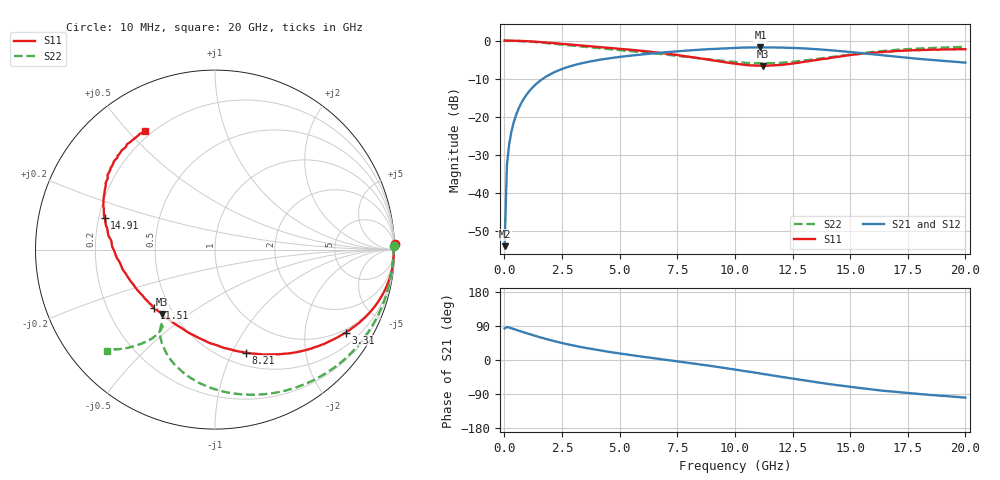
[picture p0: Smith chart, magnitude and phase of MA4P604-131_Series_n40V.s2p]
! AWR Design Environment (9226) Thu Aug 19 15:08:55 2021
! Document = 'n40V'
! nPorts: 2, nXvals: 201
# GHz S DB R 50
!Freq DBS11 AngS11 DBS21 AngS21 DBS12 AngS12 DBS22 AngS22
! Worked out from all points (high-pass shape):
!   201 points, 10 MHz to 20 GHz, reference 50 ohm
!   highest |S21| = -1.79 dB at 11.11 GHz (marker M1); lowest = -54.1 dB at 10 MHz (marker M2)
!   |S21| within 3 dB of the highest: 4.42 GHz to 17.94 GHz (13.52 GHz wide, 121 % of centre)
!   lowest |S11| = -6.7 dB at 11.21 GHz (marker M3), VSWR 2.73, Z = 21.7 - j20 ohm
!   |S11| at or under -10 dB: nowhere
!   |S22| runs from -6.0 to 0.0 dB; largest |S21 - S12| = 0.024
!   S11 on the Smith chart (normalised r, x): 10 MHz: -5, +62; 3.31 GHz: 0.89, -3.21; 8.21 GHz: 0.63, -1.13; 11.51 GHz: 0.41, -0.34; 14.91 GHz: 0.22, +0.13; 20 GHz: 0.17, +0.56
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0.01  0.02 1.8  -54.08 83.3  -52.61 73.8  -0.02 1.0
0.11  -0.04 -1.1  -32.76 87.2  -32.79 87.5  -0.06 -3.1
0.21  -0.04 -2.5  -27.19 85.5  -27.19 85.7  -0.07 -5.9
0.31  -0.04 -3.6  -23.82 83.7  -23.81 83.7  -0.08 -8.7
0.61  -0.08 -7.2  -18.01 77.6  -18.01 77.7  -0.13 -17.0
1.01  -0.18 -11.7  -13.84 69.9  -13.85 70.0  -0.26 -27.7
1.61  -0.42 -18.1  -10.30 58.8  -10.30 59.1  -0.54 -42.7
2.41  -0.82 -25.4  -7.69 46.1  -7.69 46.6  -1.01 -59.8
3.31  -1.29 -32.5  -6.03 34.3  -6.01 35.0  -1.56 -75.3
3.41  -1.34 -33.2  -5.89 33.2  -5.88 33.9  -1.61 -76.8
4.91  -2.12 -43.6  -4.38 18.1  -4.35 18.9  -2.45 -95.4
6.71  -3.20 -57.3  -3.22 3.0  -3.16 3.9  -3.50 -111.0
8.21  -4.44 -73.2  -2.52 -9.4  -2.46 -8.4  -4.53 -120.0
10.01  -6.10 -102.2  -1.93 -25.3  -1.87 -24.0  -5.68 -125.4
11.11  -6.62 -126.9  -1.79 -35.8  -1.74 -34.4  -5.99 -125.3
11.21  -6.66 -129.2  -1.79 -36.7  -1.73 -35.3  -6.00 -125.3
11.51  -6.56 -136.3  -1.80 -39.6  -1.74 -38.2  -5.97 -124.9
13.41  -5.24 -174.9  -2.23 -57.3  -2.14 -56.0  -4.96 -124.2
14.91  -3.90 164.1  -2.96 -70.1  -2.87 -68.9  -3.75 -127.3
16.71  -2.91 147.3  -4.07 -82.7  -4.01 -81.4  -2.60 -132.1
18.21  -2.46 136.1  -4.94 -90.5  -4.96 -90.0  -2.04 -135.4
20  -2.31 120.8  -5.80 -99.3  -5.97 -98.1  -1.66 -136.7
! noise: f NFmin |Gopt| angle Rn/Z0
0.01  0  1  0  2e-20
2.21  0  1  0  2e-20
4.41  0  1  0  2e-20
6.61  0  1  0  2e-20
8.81  0  1  0  2e-20
11.11  0  1  0  2e-20
13.31  0  1  0  2e-20
15.51  0  1  0  2e-20
17.71  0  1  0  2e-20
20  0  1  0  2e-20
